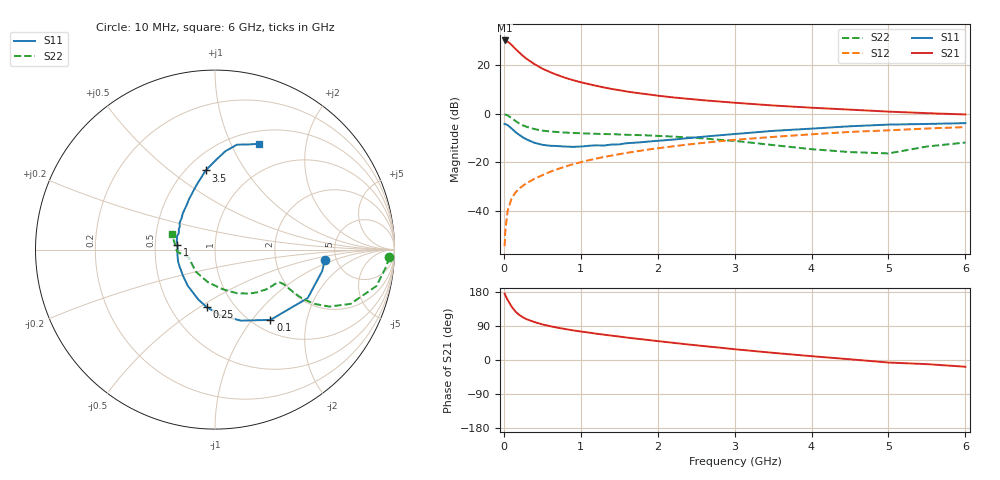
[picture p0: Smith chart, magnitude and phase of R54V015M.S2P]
! SIEMENS Small Signal Semiconductors
! BFR183
! Si NPN RF Bipolar Junction Transistor in SOT23
! VCE = 4 V  IC = 15 mA
! Common Emitter S-Parameters:  May  1996
# GHz  S  MA  R  50
!  f  S11  S21  S12  S22
! GHz  MAG  ANG  MAG  ANG  MAG  ANG  MAG  ANG
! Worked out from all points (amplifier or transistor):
!   36 points, 10 MHz to 6 GHz, reference 50 ohm
!   highest |S21| = 30.1 dB at 10 MHz (marker M1)
!   |S21| within 3 dB of that: start of sweep to 136.9 MHz
!   unconditionally stable (mu >= 1): 657.8 MHz to 2.422 GHz
!   at 250 MHz: K = 0.74, MSG = 26.6 dB, |S12| = -29.6 dB
!   at 1.4 GHz: K = 1.05, MAG = 12.4 dB, |S12| = -17.2 dB
!   at 6 GHz: K = 0.89, MSG = 2.6 dB, |S12| = -5.5 dB
!   S11 on the Smith chart (normalised r, x): 10 MHz: 4.03, -0.78; 100 MHz: 1.19, -1.24; 250 MHz: 0.75, -0.54; 1 GHz: 0.65, +0.04; 3.5 GHz: 0.62, +0.68; 6 GHz: 0.65, +1.29
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0.01  0.6147 -5.6  31.93 175.3  0.0019 90.3  0.9706 -2.5
0.02  0.6089 -11.4  31.43 170.7  0.0041 84.3  0.961 -5.3
0.05  0.583 -27.6  30.21 158.4  0.0102 77.0  0.9221 -12.7
0.1  0.4988 -51.7  25.97 141.2  0.0181 71.6  0.814 -21.8
0.15  0.4216 -69.9  21.52 128.1  0.0239 67.3  0.7115 -26.5
0.2  0.3673 -85.3  18.1 119.1  0.0289 66.2  0.6322 -28.6
0.25  0.3241 -98.0  15.31 112.4  0.0333 66.1  0.5733 -29.2
0.3  0.294 -108.3  13.25 107.3  0.0377 66.0  0.5347 -29.1
0.4  0.2518 -127.3  10.39 100.0  0.0462 67.6  0.4824 -28.2
0.5  0.2296 -141.3  8.438 94.0  0.0545 68.7  0.4493 -27.3
0.6  0.2194 -152.7  7.149 89.4  0.0639 69.1  0.4316 -26.8
0.7  0.2164 -161.9  6.198 85.2  0.0728 69.6  0.42 -26.7
0.8  0.2112 -171.2  5.449 81.6  0.0821 68.7  0.4096 -26.8
1  0.2113 172.7  4.423 75.2  0.1006 68.6  0.3964 -27.7
1.1  0.2187 167.2  4.063 72.5  0.1103 68.1  0.3912 -28.8
1.3  0.2217 155.8  3.46 66.9  0.1289 66.7  0.382 -30.6
1.6  0.2478 142.7  2.852 59.2  0.1569 64.4  0.3685 -34.5
2.2  0.2933 122.7  2.158 45.4  0.2136 58.6  0.3392 -44.3
3.5  0.4439 96.7  1.474 18.9  0.3337 42.9  0.2266 -78.3
4.5  0.5512 84.0  1.211 1.9  0.4222 30.4  0.1627 -131.3
5.5  0.6155 72.2  1.025 -10.9  0.4956 18.7  0.2119 -176.9
6  0.6393 67.2  0.964 -17.8  0.5308 11.1  0.2555 159.9
